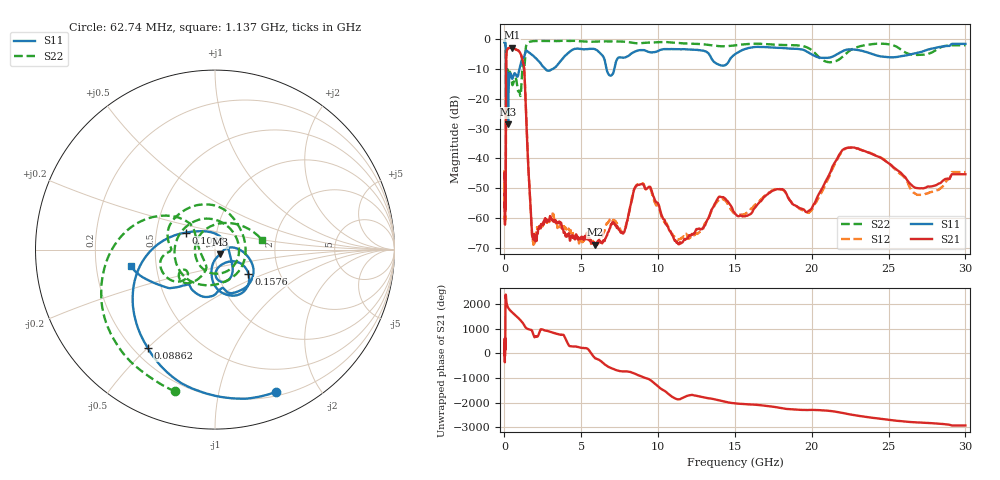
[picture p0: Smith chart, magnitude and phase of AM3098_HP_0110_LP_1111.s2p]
! Date/Time: Thu, Feb 28, 2019 8:38 AM
! Network Analyzer: Agilent Technologies E8364B Rev: A.07.50.67
! Sweep from 0.010 to 30.000 GHz, 1601 Points, Sweep Type: LOG
! Power Supply: 5.022 V, 0.002 A
# Hz S DB R 50
!freq MagS11 AngS11 MagS21 AngS21 MagS12 AngS12 MagS22 AngS22
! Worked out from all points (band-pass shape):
!   1601 points, 10 MHz to 30 GHz, reference 50 ohm
!   highest |S21| = -2.76 dB at 498 MHz (marker M1); lowest = -69.0 dB at 5.9 GHz (marker M2)
!   |S21| within 3 dB of the highest: 118.9 MHz to 1.113 GHz (994.3 MHz wide, 161 % of centre)
!   lowest |S11| = -28.6 dB at 236.3 MHz (marker M3), VSWR 1.08, Z = 52.7 - j2.7 ohm
!   |S11| at or under -10 dB: 99.94 MHz to 973.1 MHz (873.1 MHz wide, 163 % of centre); 2.67 GHz to 3.129 GHz (458.6 MHz wide, 15.8 % of centre); 6.644 GHz to 7.151 GHz (507 MHz wide, 7.35 % of centre)
!   |S22| runs from -21.9 to -0.5 dB; largest |S21 - S12| = 0.011
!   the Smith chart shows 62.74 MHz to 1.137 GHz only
!   S11 on the Smith chart (normalised r, x): 62.74 MHz: 0.24, -1.49; 88.62 MHz: 0.26, -0.50; 102.5 MHz: 0.71, +0.14; 157.6 MHz: 1.39, -0.39; 1.137 GHz: 0.36, -0.09
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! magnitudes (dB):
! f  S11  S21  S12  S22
! 10 MHz  -0.4  -46.4  -45.6  -0.6
! 38.04 MHz  -0.5  -59.9  -56.4  -1.0
! 62.74 MHz  -1.3  -53.4  -52.3  -1.7
! 88.62 MHz  -3.6  -44.1  -43.0  -3.8
! 102.5 MHz  -14.5  -14.7  -14.7  -19.0
! 144.7 MHz  -18.6  -3.9  -3.8  -14.0
! 157.6 MHz  -12.8  -3.6  -3.6  -11.8
! 236.3 MHz  -28.6  -3.0  -2.9  -11.9
! 311.2 MHz  -12.6  -2.9  -2.8  -11.2
! 498 MHz  -13.2  -2.8  -2.7  -15.0
! 550.5 MHz  -12.7  -2.9  -2.9  -15.1
! 1.137 GHz  -6.4  -6.2  -6.2  -11.4
! 1.308 GHz  -5.4  -12.2  -12.1  -8.9
! 1.811 GHz  -5.3  -66.0  -66.7  -0.6
! 2.084 GHz  -6.5  -67.5  -64.6  -0.5
! 5.9 GHz  -3.3  -69.0  -69.5  -0.7
! 7.926 GHz  -5.9  -62.5  -62.1  -0.8
! 8.804 GHz  -3.6  -48.8  -48.4  -1.3
! 11.42 GHz  -3.3  -68.1  -67.0  -1.2
! 19.61 GHz  -3.9  -58.0  -58.0  -2.5
! 22.67 GHz  -3.4  -36.3  -36.5  -3.2
! 30 GHz  -1.5  -45.3  -44.6  -2.0
